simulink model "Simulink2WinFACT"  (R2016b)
settings: Solver=ode3  StartTime=0.0  StopTime=600  FixedStep=0.01  RelTol=1e-3  EnableMultiTasking=on
libraries: instrumentlib x1

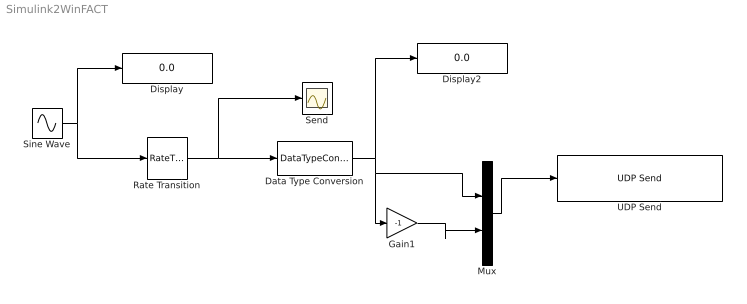
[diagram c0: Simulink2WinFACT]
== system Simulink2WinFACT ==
  Data Type Conversion : DataTypeConversion  OutDataTypeStr=double
  Display : Display
  Display2 : Display
  Gain1 : Gain  Gain=-1
  Mux : Mux  Inputs=2
  Rate Transition : RateTransition  OutPortSampleTimeOpt=Inherit
  Send : Scope
  Sine Wave : Sin  Frequency=0.1  SampleTime=0
  UDP Send : instrumentlib/UDP Send  Priority=1  Host=127.0.0.1  Port=1600  LocalPort=-1  EnableBlockingMode=on  ByteOrder=LittleEndian
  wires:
  Sine Wave/1 -> Display/1, Rate Transition/1
  Rate Transition/1 -> Data Type Conversion/1, Send/1
  Data Type Conversion/1 -> Gain1/1, Mux/1, Display2/1
  Mux/1 -> UDP Send/1
  Gain1/1 -> Mux/2
